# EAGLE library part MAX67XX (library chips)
A simple watchdog timer with adjustable timeouts and reset time
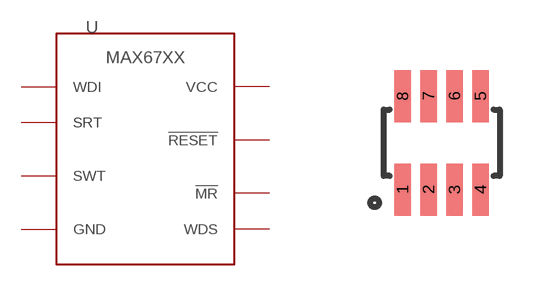
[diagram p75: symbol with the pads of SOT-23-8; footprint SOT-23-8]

Designator prefix U

## MAX67XXMAX6746MAX67XX (DIGIKEY: MAX6746KA26+TCT-ND; MANUFACTURER: Maxim Integrated; MPN: MAX6746KA26+T), MAX67XXMAX6749MAX67XX (DIGIKEY: MAX6749KA+TCT-ND; MANUFACTURER: Maxim Integrated; MPN: MAX6749KA+T)  [SOT-23-8]
1  !MR
2  SWT
3  SRT
4  GND
5  WDS
6  WDI
7  !RESET
8  VCC

## Footprint SOT-23-8 (pad centres in mm)
smd 0.42 x 1.3: 1 -0.975,-1.17; 2 -0.325,-1.17; 3 0.325,-1.17; 4 0.975,-1.17; 5 0.975,1.17; 6 0.325,1.17; 7 -0.325,1.17; 8 -0.975,1.17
